(* Logix 5000 AddOnInstructionDefinition export AMCI_NXFE2_Immediate_Stop; software revision 20.03 *)

ADD_ON_INSTRUCTION AMCI_NXFE2_Immediate_Stop   (* revision 1.1, vendor AMCI *)
// Revision note:
// Version 1.1 added the slot_axis number and the input parameters can now be tags or discrete values.
VAR_IN_OUT
   NXFE2_output_data : _000A:NXFE2_0986AEB4:O:0; {required}
END_VAR
VAR
   command_data_block : INT[10];
        [0]   // Command Bits MSW
        [1]   // Command Bits LSW
        [2]   // Upper Target Position
        [3]   // Lower Target Position
        [4]   // Upper Programmed Speed
        [5]   // Lower Programmed Speed
END_VAR

ROUTINE Logic   (* ladder *)
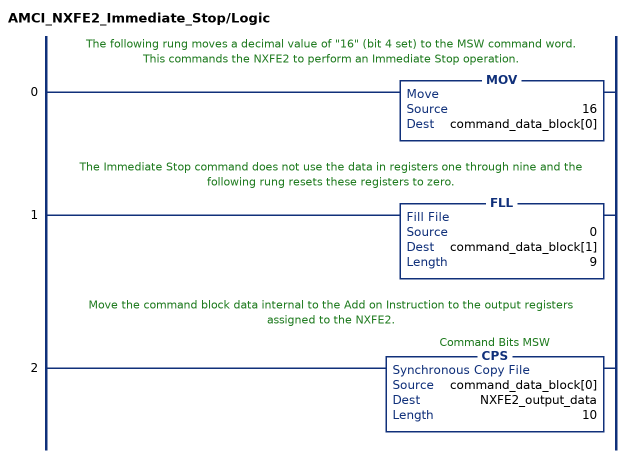
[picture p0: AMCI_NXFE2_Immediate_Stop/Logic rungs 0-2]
   // The following rung moves a decimal value of "16" (bit 4 set) to the MSW command word.  This commands the NXFE2 to perform an Immediate Stop operation.
   0: MOV(16,command_data_block[0]);
   // The Immediate Stop command does not use the data in registers one through nine and the following rung resets these registers to zero.
   1: FLL(0,command_data_block[1],9);
   // Move the command block data internal to the Add on Instruction to the output registers assigned to the NXFE2.
   2: CPS(command_data_block[0],NXFE2_output_data,10);
END_ROUTINE
END_ADD_ON_INSTRUCTION
